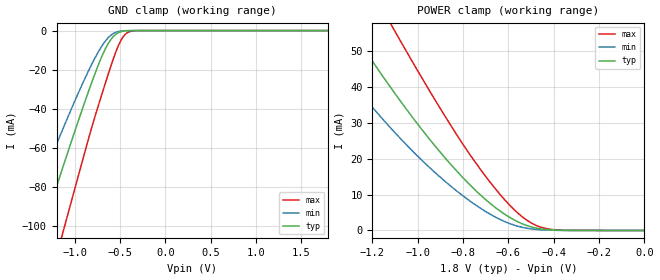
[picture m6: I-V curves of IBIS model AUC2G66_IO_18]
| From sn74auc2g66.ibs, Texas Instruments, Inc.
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[Model]   AUC2G66_IO_18
Model_type  Terminator
| variable   typ   min   max
C_comp   3.59pF   3.21pF   3.74pF
| C_tri-state   3.59pF   3.21pF   3.74pF
[Temperature Range]   40   100   -40
| Ambient temperature   25   85   -40
[Voltage range]   1.8   1.65   1.95
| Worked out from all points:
|   GND clamp passes 1 mA (typ) near -0.51 V on its own axis
|   POWER clamp passes 1 mA (typ) near -0.50 V on its own axis
[GND Clamp]
| AUC2G66_IO_18
|   Voltage   I(typ)   I(min)   I(max)
-2.7V     -295.9mA   -240.2mA   -365.2mA
-1.595V   -136.6mA   -104.5mA   -182mA
-1.55V    -130.1mA   -99.12mA   -174.5mA
-1.345V   -100.6mA   -74.92mA   -140mA
-1.135V   -70.7mA    -50.96mA   -104.3mA
-1.105V   -66.47mA   -47.63mA   -99.21mA
-750mV    -18.95mA   -11.84mA   -40.11mA
-650mV    -8.356mA   -4.727mA   -25.29mA
-560mV    -2.479mA   -1.155mA   -12.74mA
-460mV    -288.2uA   -115.8uA   -2.895mA
-355mV    -15.11uA   -7.432uA   -159.4uA
1.8V      503.3pA    46.32nA    420.5pA
[POWER Clamp]
| AUC2G66_IO_18
|   Voltage   I(typ)   I(min)   I(max)
-2.7V     214.4mA    184.8mA    244.7mA
-1.47V    73.54mA    55.84mA    97.67mA
-1.3V     56.54mA    41.83mA    77.93mA
-1.115V   39.34mA    28.17mA    56.97mA
-1.095V   37.58mA    26.81mA    54.75mA
-930mV    23.98mA    16.46mA    36.95mA
-780mV    13.32mA    8.657mA    22.02mA
-635mV    5.323mA    3.01mA     9.881mA
-535mV    1.766mA    822.1uA    3.615mA
-475mV    637.7uA    272.6uA    1.344mA
-395mV    100.5uA    45.32uA    191.6uA
-35.59fV  503.3pA    841.7pA    502.9pA
